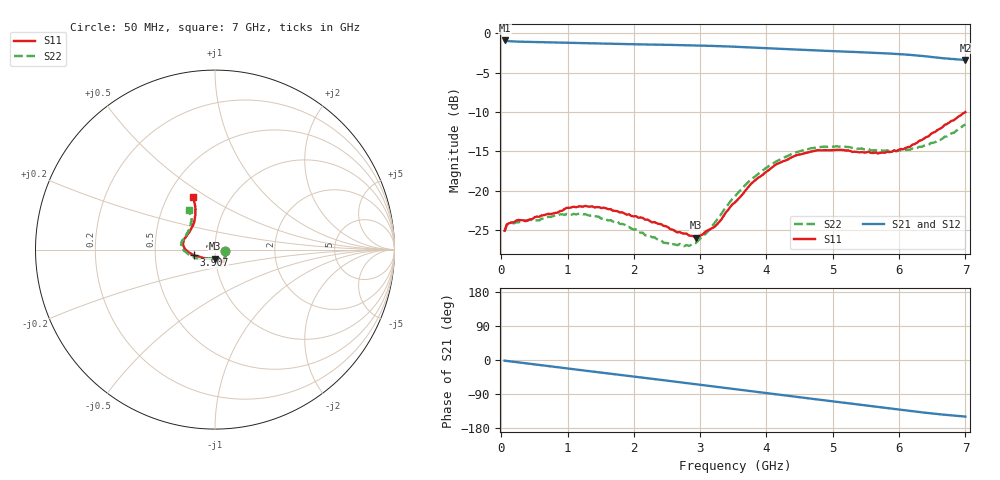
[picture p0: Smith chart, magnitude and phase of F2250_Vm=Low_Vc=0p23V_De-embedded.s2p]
! Integrated Device Technology
! Corporate Headquarters
! 6024 Silver Creek Valley Road
! San Jose, CA 95138  USA
! Phone:  1-408-284-8200
! Toll Free:  1-800-223-1366
! Webpage:  http://www.idt.com/
! Timing and RF Division
! 515 Groton Road, Suite 102
! Westford, MA 01886-6024
! Device:  F2250
! Description: Voltage Variable RF Attenuator
! Frequency:  50.0 -  6000.00 MHz
! Package:  3x3 mm Thin QFN Plastic Package: 16 pin
! Ports:  2 RF, 3 DC
!  Pin  1  = GND
!  Pin  2  = NC
!  Pin  3  = RF1  = Port 1
!  Pin  4  = NC
!  Pin  5  = GND
!  Pin  6  = GND
!  Pin  7  = GND
!  Pin  8  = GND
!  Pin  9  = NC
!  Pin 10  = RF2  = Port 2
!  Pin 11  = NC
!  Pin 12  = GND
!  Pin 13  = GND
!  Pin 14  = VCNTRL
!  Pin 15  = VDD
!  Pin 16  = VMODE
! Vcntrl:  0.230 Volts
! Vmode:  +0.000 Volts
! Vdd:  +3.30  Volts
! Current:  1.106 mA
! Data:  The device was measured on a the F2250 evaluation board which has
!  individual transmission lines to the RF pins.  Data was collected
!  using a calibrated network analyzer.  The evaluation board was
!  de-embedded using a TRL calibration technique.
!  The reference plane is the edge of the package pin.
! Misc:  SN 10
!  Action Tracker AT0258
! Date Measured:  2014-11-26
! Date:  2015-10-15  MJV
! Note:
!  Integrated Device Technology supplies this data as a sample of measured
!  data at the package pin for this product.  Your particular data for this
!  product may vary.
!  Data was taken at 25 degrees C.
!  Integrated Device Technology reserves the right to change this data at anytime.
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# GHz S dB R 50
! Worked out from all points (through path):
!   201 points, 50 MHz to 7 GHz, reference 50 ohm
!   highest |S21| = -0.93 dB at 50 MHz (marker M1); lowest = -3.4 dB at 7 GHz (marker M2)
!   group delay of S21, straight-line fit = 60 ps
!   lowest |S11| = -25.9 dB at 2.934 GHz (marker M3), VSWR 1.11, Z = 49.6 - j5.02 ohm
!   |S11| at or under -10 dB: start of sweep to end of sweep
!   |S22| runs from -27.0 to -11.6 dB; largest |S21 - S12| = 0.00033
!   S11 on the Smith chart (normalised r, x): 50 MHz: 1.12, -0.02; 3.907 GHz: 0.79, -0.05; 7 GHz: 0.67, +0.43
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0.05  -25.06 -9.7  -0.93 -1.8  -0.93 -1.8  -25.18 -10.1
0.08475  -24.24 -9.6  -1.00 -2.5  -1.00 -2.5  -24.29 -9.4
0.15425  -24.01 -11.8  -1.04 -4.0  -1.04 -4.0  -24.06 -11.0
0.57125  -23.30 -30.0  -1.15 -13.1  -1.14 -13.1  -23.77 -30.4
0.884  -22.58 -45.7  -1.21 -19.9  -1.21 -19.9  -23.00 -46.8
1.2315  -22.02 -55.9  -1.28 -27.4  -1.28 -27.4  -23.01 -59.6
1.75275  -22.58 -62.6  -1.38 -38.4  -1.38 -38.4  -23.90 -66.6
2.37825  -24.21 -63.4  -1.47 -51.8  -1.47 -51.8  -26.23 -67.8
2.552  -24.89 -67.6  -1.49 -55.6  -1.49 -55.6  -26.88 -73.5
2.83  -25.67 -83.0  -1.55 -61.7  -1.54 -61.7  -27.00 -92.7
2.93425  -25.93 -92.1  -1.57 -64.0  -1.56 -64.0  -26.63 -101.5
3.21225  -24.60 -121.8  -1.63 -70.1  -1.63 -70.1  -24.13 -127.5
3.525  -21.48 -148.1  -1.73 -77.1  -1.72 -77.1  -20.70 -146.4
3.76825  -19.11 -161.2  -1.82 -82.5  -1.81 -82.5  -18.54 -156.7
3.90725  -18.19 -165.5  -1.87 -85.5  -1.87 -85.5  -17.65 -162.8
4.1505  -16.62 -173.6  -1.97 -90.8  -1.97 -90.8  -16.26 -171.4
4.7065  -14.97 172.3  -2.18 -102.8  -2.18 -102.8  -14.59 175.7
5.15825  -14.83 161.5  -2.34 -112.5  -2.34 -112.5  -14.35 166.5
5.85325  -15.09 138.4  -2.59 -127.5  -2.59 -127.5  -14.97 151.5
6.166  -14.41 127.6  -2.76 -134.3  -2.76 -134.3  -14.79 142.6
6.444  -13.10 119.3  -2.97 -140.1  -2.97 -140.1  -14.17 133.3
7  -10.02 113.0  -3.41 -149.4  -3.41 -149.4  -11.59 123.8
